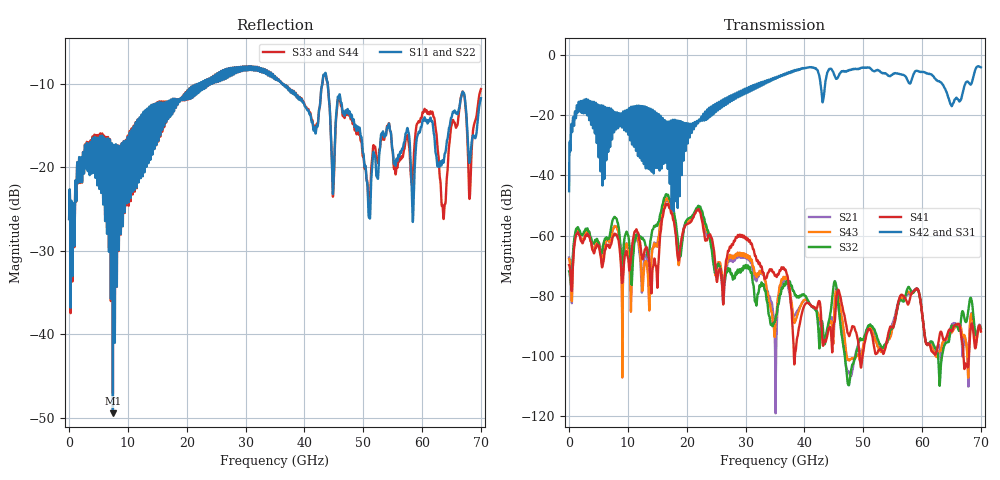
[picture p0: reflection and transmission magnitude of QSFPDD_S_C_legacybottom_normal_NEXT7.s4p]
! AWR Design Environment (8415) Thu Dec 20 14:55:38 2018
! Document = 'CHANNEL TEST'
! nPorts: 4, nXvals: 7001
# HZ S DB R 50
!Freq DBS11 AngS11 DBS12 AngS12 DBS13 AngS13 DBS14 AngS14
!	DBS21 AngS21 DBS22 AngS22 DBS23 AngS23 DBS24 AngS24
!	DBS31 AngS31 DBS32 AngS32 DBS33 AngS33 DBS34 AngS34
!	DBS41 AngS41 DBS42 AngS42 DBS43 AngS43 DBS44 AngS44
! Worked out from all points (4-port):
!   7000 points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, 10 MHz to 70 GHz, reference 50 ohm
!   strongest paths, dB at 10 MHz, 17.51 GHz, 35.01 GHz, 52.51 GHz, 70 GHz:
!     S42: -45.2, -28.8, -7.5, -5.0, -4.0
!     S31: -45.3, -28.7, -7.5, -5.0, -4.0
!     S41: -69.8, -52.8, -73.3, -98.4, -91.9
!     S32: -71.9, -49.8, -88.5, -94.6, -90.8
!     S43: -67.8, -51.1, -91.9, -97.0, -91.7
!     S21: -67.3, -51.5, -97.5, -96.3, -90.9
!   lowest |S11| = -49.4 dB at 7.45 GHz (marker M1), VSWR 1.01, Z = 50.3 + j0.0931 ohm
!   |S11| at or under -10 dB: start of sweep to 22.1 GHz; 36.25 GHz to 43.06 GHz (6.813 GHz wide, 17.2 % of centre); 43.96 GHz to end of sweep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
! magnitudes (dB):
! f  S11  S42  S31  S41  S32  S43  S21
! 10 MHz  -26.2  -45.2  -45.3  -69.8  -71.9  -67.8  -67.3
! 1.64 GHz  -19.9  -15.5  -15.5  -59.6  -57.9  -58.4  -58.4
! 7.45 GHz  -49.4  -18.5  -18.5  -60.4  -54.6  -58.0  -57.9
! 13.58 GHz  -15.3  -18.1  -18.1  -67.7  -66.0  -81.9  -74.4
! 22.13 GHz  -9.9  -21.4  -21.4  -51.9  -50.4  -51.3  -51.4
! 31.82 GHz  -8.4  -10.1  -10.1  -67.8  -83.2  -73.6  -75.0
! 70 GHz  -11.8  -4.0  -4.0  -91.9  -90.8  -91.7  -90.9
